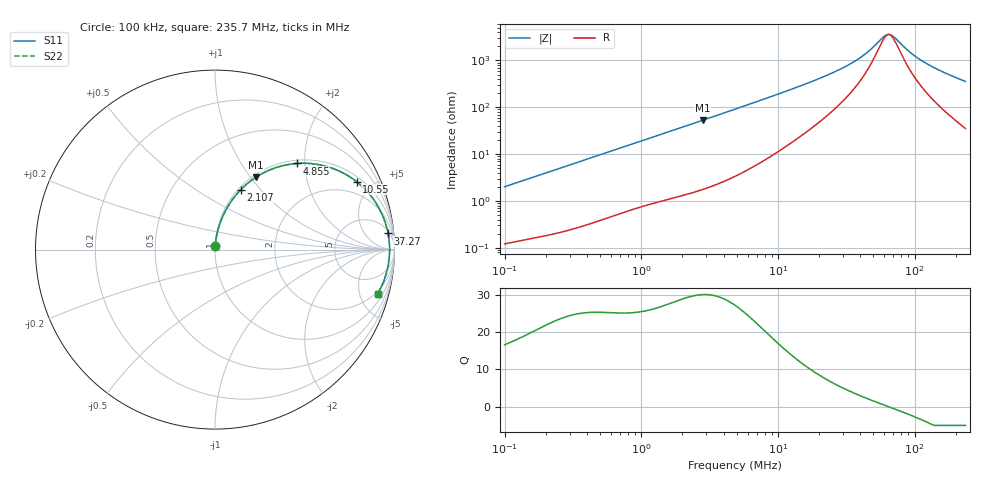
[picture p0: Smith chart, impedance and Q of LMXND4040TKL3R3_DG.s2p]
! LMXND4040TKL3R3_DG  S-PARAMETER MODEL  ( General Type )
! Model Generated by TAIYO YUDEN Corporation (http://www.ty-top.com)
! Version 1.0
! TAIYO YUDEN Control No. 191023NI43SB-FBB
! Copyright(c) 2019 TAIYO YUDEN CO.,LTD. All Rights Reserved.
! Product Description (link to TY-COMPAS)
! https://ds.yuden.co.jp/TYCOMPAS/or/detail?pn=LMXND4040TKL3R3MDG&u=M
! Products Name : Inductors
! Characteristics :
!  Inductance : 3.3 uH , SRF(min) : 45 MHz , DC Resistance(max) : 0.066 Ohm
!  Rated Current : Saturation :2300 mA , Temp Rise : 2000 mA
!  Case Size : 4.0 x 4.0 / 0.157 x 0.157 [mm/inch] , Thickness : 1.8 / 0.071 [mm/inch]
!  (Conditions: Temperature = 25 degC , DC Bias Current/Voltage = 0A / 0V)
! External Node Assignments :
!  1  o---GGG---o  2
! GND o---------o GND
! Frequency Range : 0.1MHz  -  235.669543MHz  [ 402 STEP ]
# MHz S RI R 50
! Freq[MHz].  S11 Real  S11 Imag  S21 Real  S21 Imag  S12 Real  S12 Imag  S22 Real  S22 Imag
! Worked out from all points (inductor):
!   401 points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, 100 kHz to 235.7 MHz, reference 50 ohm
!   read as one part in series: L = 3.18 uH near 104 kHz
!   highest Q = 30 at 2.819 MHz (marker M1), where L = 2.98 uH
!   self-resonance near 64.71 MHz
!   S11 on the Smith chart (normalised r, x): 100 kHz: 1.00, +0.04; 2.107 MHz: 1.03, +0.79; 4.855 MHz: 1.07, +1.82; 10.55 MHz: 1.25, +4.03; 37.27 MHz: 7, +19; 235.7 MHz: 1.71, -7.09
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0.1  0.00161 0.02  0.9984 -0.02  0.9984 -0.02  0.00161 0.02
0.367165  0.00794 0.071  0.9921 -0.071  0.9921 -0.071  0.00794 0.071
0.73853  0.0251 0.1378  0.9749 -0.1378  0.9749 -0.1378  0.0251 0.1378
1.348099  0.0691 0.2356  0.9309 -0.2356  0.9309 -0.2356  0.0691 0.2356
2.106828  0.1442 0.3345  0.8558 -0.3345  0.8558 -0.3345  0.1442 0.3345
2.81897  0.2262 0.402  0.7738 -0.402  0.7738 -0.402  0.2262 0.402
3.771828  0.3386 0.4565  0.6614 -0.4565  0.6614 -0.4565  0.3386 0.4565
4.854581  0.4552 0.4799  0.5448 -0.4799  0.5448 -0.4799  0.4552 0.4799
6.885023  0.6222 0.4632  0.3778 -0.4632  0.3778 -0.4632  0.6222 0.4632
10.55315  0.7886 0.3786  0.2114 -0.3786  0.2114 -0.3786  0.7886 0.3786
17.8243  0.9058 0.2449  0.0942 -0.2449  0.0942 -0.2449  0.9058 0.2449
27.32054  0.9492 0.149  0.0508 -0.149  0.0508 -0.149  0.9492 0.149
37.27189  0.9643 0.0902  0.0357 -0.0902  0.0357 -0.0902  0.9643 0.0902
46.14448  0.9698 0.0539  0.0302 -0.0539  0.0302 -0.0539  0.9698 0.0539
59.39086  0.9727 0.0135  0.0273 -0.0135  0.0273 -0.0135  0.9727 0.0135
62.95234  0.9729 0.00431  0.0271 -0.00431  0.0271 -0.00431  0.9729 0.00431
65.44454  0.9729 -0.00178  0.0271 0.00178  0.0271 0.00178  0.9729 -0.00178
70.72882  0.9727 -0.014  0.0273 0.014  0.0273 0.014  0.9727 -0.014
92.8169  0.9695 -0.0577  0.0305 0.0577  0.0305 0.0577  0.9695 -0.0577
117.1645  0.963 -0.0978  0.037 0.0978  0.037 0.0978  0.963 -0.0978
162.9743  0.9452 -0.1618  0.0548 0.1618  0.0548 0.1618  0.9452 -0.1618
235.6695  0.906 -0.2462  0.094 0.2462  0.094 0.2462  0.906 -0.2462
